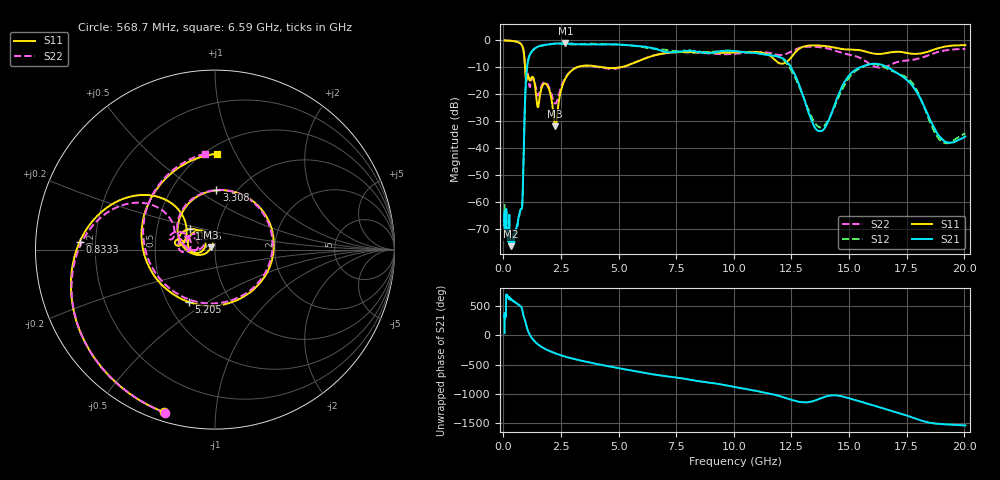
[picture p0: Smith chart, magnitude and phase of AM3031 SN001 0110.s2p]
# Hz S DB R 50
!freq MagS11 AngS11 MagS21 AngS21 MagS12 AngS12 MagS22 AngS22
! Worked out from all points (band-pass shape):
!   1601 points, 50 MHz to 20.05 GHz, reference 50 ohm
!   highest |S21| = -1.07 dB at 2.692 GHz (marker M1); lowest = -76.4 dB at 329.1 MHz (marker M2)
!   |S21| within 3 dB of the highest: 1.238 GHz to 6.936 GHz (5.698 GHz wide, 139 % of centre); 9.392 GHz to 10.18 GHz (786 MHz wide, 8.03 % of centre)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
!   lowest |S11| = -31.9 dB at 2.249 GHz (marker M3), VSWR 1.05, Z = 47.9 + j1.32 ohm
!   |S11| at or under -10 dB: 937.3 MHz to 3.172 GHz (2.235 GHz wide, 109 % of centre); 4.367 GHz to 5.036 GHz (668.7 MHz wide, 14.2 % of centre)
!   |S22| runs from -23.5 to 0.0 dB; largest |S21 - S12| = 0.067
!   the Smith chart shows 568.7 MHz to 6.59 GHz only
!   S11 on the Smith chart (normalised r, x): 568.7 MHz: 0.04, -0.73; 833.3 MHz: 0.14, +0.03; 1.326 GHz: 0.74, +0.17; 3.308 GHz: 0.81, +0.60; 5.205 GHz: 0.64, -0.42; 6.59 GHz: 0.56, +0.85
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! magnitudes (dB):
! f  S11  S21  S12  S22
! 50 MHz  0.0  -67.1  -60.8  0.0
! 135.9 MHz  0.0  -70.5  -70.1  0.0
! 252.2 MHz  -0.1  -65.2  -65.1  -0.1
! 329.1 MHz  -0.1  -76.4  -76.0  -0.1
! 369.6 MHz  -0.2  -74.6  -75.0  -0.2
! 568.7 MHz  -0.5  -69.4  -69.3  -0.4
! 833.3 MHz  -2.4  -57.5  -57.5  -2.5
! 1.005 GHz  -14.8  -11.4  -11.3  -11.8
! 1.326 GHz  -14.8  -3.2  -3.3  -14.4
! 1.495 GHz  -24.8  -2.3  -2.3  -20.4
! 1.914 GHz  -16.8  -1.6  -1.6  -16.3
! 2.249 GHz  -31.9  -1.1  -1.2  -23.5
! 2.692 GHz  -14.0  -1.1  -1.3  -13.7
! 2.722 GHz  -13.6  -1.1  -1.3  -13.3
! 3.308 GHz  -9.6  -1.4  -1.4  -9.7
! 5.205 GHz  -9.7  -1.6  -1.6  -9.9
! 6.59 GHz  -5.4  -3.1  -3.0  -5.4
! 7.402 GHz  -4.4  -4.3  -3.9  -4.4
! 11.91 GHz  -8.2  -6.0  -6.0  -5.3
! 13.73 GHz  -1.9  -33.7  -32.3  -2.5
! 16.32 GHz  -5.0  -8.8  -9.2  -10.1
! 20.05 GHz  -1.8  -35.7  -34.5  -3.1
